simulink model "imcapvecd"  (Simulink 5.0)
settings: Solver=ode45  StartTime=0  StopTime=12.7  MaxStep=5e-4  RelTol=1e-4
libraries: simulink x3

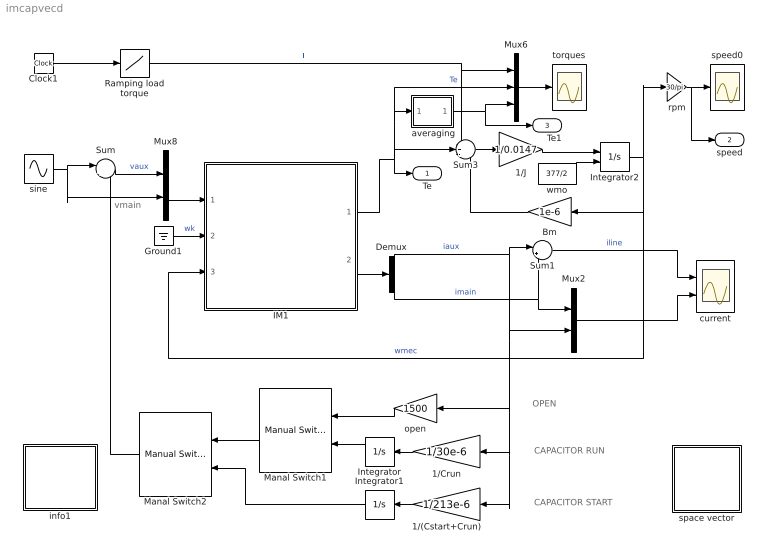
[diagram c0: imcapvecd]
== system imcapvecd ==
  note: OPEN
  note: CAPACITOR RUN
  note: CAPACITOR START
  note: vmain
  " averaging" : Subsystem
  1/(Cstart+Crun) : Gain  Orientation=left  Gain=1/213e-6
  1/Crun : Gain  Orientation=left  Gain=1/30e-6
  1/J : Gain  Gain=1/0.0147
  Bm : Gain  Orientation=left  Gain=1e-6
  Clock1 : Clock
  Demux : Demux  Outputs=2
  Ground1 : Ground
  IM1 : Subsystem  mask(Inductionmachine){Rs=2.02, Rr=4.12, Lsl=8.54e-3, Lrl=3.13e-3, Lm=180e-3, wo=2*pi*60, p=4}
      mask prompts: Rs "Stator resistance [ohm]"; Rr "Rotor resistance [ohm]"; Lsl "Stator leakage inductance  [H]"; Lrl "Rotor leakage inductance [H]"; Lm "Magnetizing inductance [H]"; wo "Base frequency [rad/s]"; p "Number of poles"
      mask help: Space vector model of the induction machine in a general frame k. SI units
  Integrator : Integrator  Orientation=left
  Integrator1 : Integrator  Orientation=left
  Integrator2 : Integrator  InitialConditionSource=external  InitialCondition=377/2
  Manal Switch1 : simulink/Signal Routing/Manual Switch  Orientation=left  sw=0  action=0
  Manal Switch2 : simulink/Signal Routing/Manual Switch  Orientation=left  sw=0  action=0
  Mux2 : Mux  Inputs=2
  Mux6 : Mux  Inputs=3
  Mux8 : Mux  Inputs=2
  Ramping load torque : Lookup  InputValues=[0 .5 5]  OutputValues=[0 0 3.50]
  Sum : Sum  Inputs=|+-
  Sum1 : Sum  Inputs=|++
  Sum3 : Sum  Inputs=-+-
  current : Scope  NumInputPorts=2
  info1 : Subsystem
  open : Gain  Orientation=left  Gain=1500
  rpm : Gain  Gain=30/pi
  sine : Sin  Amplitude=110*sqrt(2)  Frequency=2*pi*60  Phase=pi/2  SampleTime=0
  space vector : Subsystem
  speed0 : Scope
  torques : Scope
  wmo : Constant  Value=377/2
  Te : Outport
  speed : Outport  Port=2
  Te1 : Outport  Port=3
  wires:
  Sum1/1 -> current/1  "iline"
  Mux2/1 -> current/2
  Mux8/1 -> IM1/1(vs)
  Sum/1 -> Mux8/1  "vaux"
  sine/1 -> Mux8/2, Sum/1
  IM1/2(is) -> Demux/1
  Demux/1 -> Sum1/1, Mux2/2, open/1, 1/(Cstart+Crun)/1, 1/Crun/1  "iaux"
  Demux/2 -> Sum1/2, Mux2/1  "imain"
  1/J/1 -> Integrator2/1
  Mux6/1 -> torques/1
  Bm/1 -> Sum3/3
  Integrator2/1 -> Bm/1, IM1/3(wmec), rpm/1  "wmec"
  rpm/1 -> speed/1, speed0/1
  IM1/1(Te) -> Sum3/2, Te/1, Mux6/2, " averaging"/1(sig)  "Te"
  Sum3/1 -> 1/J/1
  Clock1/1 -> Ramping load torque/1
  Ramping load torque/1 -> Mux6/1, Sum3/1  "Tl"
  Ground1/1 -> IM1/2(wk)  "wk"
  " averaging"/1(ave) -> Mux6/3, Te1/1
  open/1 -> Manal Switch1/1
  Integrator/1 -> Manal Switch1/2
  1/Crun/1 -> Integrator/1
  Manal Switch1/1 -> Manal Switch2/1
  Manal Switch2/1 -> Sum/2
  1/(Cstart+Crun)/1 -> Integrator1/1
  Integrator1/1 -> Manal Switch2/2
  wmo/1 -> Integrator2/2

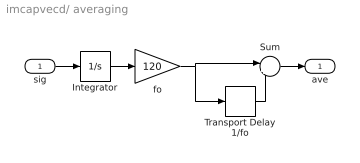
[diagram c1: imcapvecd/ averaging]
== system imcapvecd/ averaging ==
  sig : Inport
  Integrator : Integrator
  Sum : Sum  Inputs=|+-
  Transport Delay 1/fo : TransportDelay  DelayTime=1/120
  fo : Gain  Gain=120
  ave : Outport
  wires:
  Sum/1 -> ave/1
  Transport Delay 1/fo/1 -> Sum/2
  sig/1 -> Integrator/1
  fo/1 -> Transport Delay 1/fo/1, Sum/1
  Integrator/1 -> fo/1

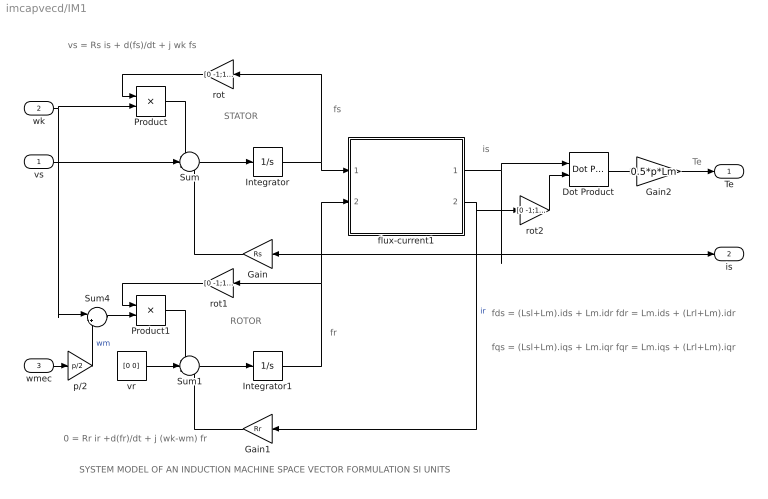
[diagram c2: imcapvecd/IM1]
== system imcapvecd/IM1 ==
  note: ROTOR
  note: STATOR
  note: fs
  note: is
  note: Te
  note: SYSTEM MODEL OF AN INDUCTION MACHINE SPACE VECTOR FORMULATION SI UNITS
  note: vs = Rs is + d(fs)/dt + j wk fs
  note: 0 = Rr ir +d(fr)/dt + j (wk-wm) fr
  note: fds = (Lsl+Lm).ids + Lm.idr fdr = Lm.ids + (Lrl+Lm).idr
  note: fqs = (Lsl+Lm).iqs + Lm.iqr fqr = Lm.iqs + (Lrl+Lm).iqr
  note: fr
  vs : Inport
  wk : Inport  Port=2
  wmec : Inport  Port=3
  Dot Product : simulink/Math Operations/Dot Product
  Gain : Gain  Orientation=left  Gain=Rs
  Gain1 : Gain  Orientation=left  Gain=Rr
  Gain2 : Gain  Gain=0.5*p*Lm
  Integrator : Integrator  InitialCondition=[0 0]
  Integrator1 : Integrator  InitialCondition=[0 0]
  Product : Product
  Product1 : Product
  Sum : Sum  Inputs=-+-
  Sum1 : Sum  Inputs=-+-
  Sum4 : Sum  Inputs=|+-
  flux-current1 : Subsystem
  p/2 : Gain  Gain=p/2
  rot : Gain  Orientation=left  Gain=[0 -1;1 0]  Multiplication=Matrix(K*u)
  rot1 : Gain  Orientation=left  Gain=[0 -1;1 0]  Multiplication=Matrix(K*u)
  rot2 : Gain  Gain=[0 -1;1 0]  Multiplication=Matrix(K*u)
  vr : Constant  Value=[0 0]
  Te : Outport
  is : Outport  Port=2
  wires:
  Gain/1 -> Sum/3
  vr/1 -> Sum1/2
  Gain1/1 -> Sum1/3
  Integrator/1 -> flux-current1/1(fs), rot/1
  Integrator1/1 -> rot1/1, flux-current1/2(fr)
  Product1/1 -> Sum1/1
  rot1/1 -> Product1/1
  Product/1 -> Sum/1
  rot/1 -> Product/1
  Sum4/1 -> Product1/2
  vs/1 -> Sum/2
  wk/1 -> Product/2, Sum4/1
  Sum1/1 -> Integrator1/1
  Sum/1 -> Integrator/1
  flux-current1/1(is) -> Gain/1, is/1, Dot Product/1
  Dot Product/1 -> Gain2/1
  Gain2/1 -> Te/1
  wmec/1 -> p/2/1
  p/2/1 -> Sum4/2  "wm"
  rot2/1 -> Dot Product/2
  flux-current1/2(ir) -> Gain1/1, rot2/1  "ir"

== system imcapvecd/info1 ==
  note: Three configurations can be studied: A) Single phase (stop time = 6s) B) Capacitor run (stop time = 7s) C) Capacitor start (stop time =12.7s)
  note: Quasi-static characteristics of a single-phase capacitor induction motor:

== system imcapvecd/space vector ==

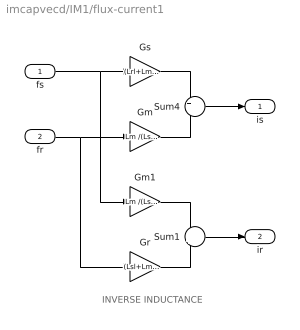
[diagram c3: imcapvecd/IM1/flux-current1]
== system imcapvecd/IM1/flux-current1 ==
  note: INVERSE INDUCTANCE
  fs : Inport
  fr : Inport  Port=2
  Gm : Gain  Gain=Lm /(Lsl*Lrl+Lsl*Lm+Lrl*Lm)
  Gm1 : Gain  Gain=Lm /(Lsl*Lrl+Lsl*Lm+Lrl*Lm)
  Gr : Gain  Gain=(Lsl+Lm )/(Lsl*Lrl+Lsl*Lm+Lrl*Lm)
  Gs : Gain  Gain=(Lrl+Lm) /(Lsl*Lrl+Lsl*Lm+Lrl*Lm)
  Sum1 : Sum  Inputs=-+
  Sum4 : Sum  Inputs=+-
  is : Outport
  ir : Outport  Port=2
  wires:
  fs/1 -> Gs/1, Gm1/1
  Gs/1 -> Sum4/1
  fr/1 -> Gm/1, Gr/1
  Gm/1 -> Sum4/2
  Sum4/1 -> is/1
  Gm1/1 -> Sum1/1
  Gr/1 -> Sum1/2
  Sum1/1 -> ir/1
